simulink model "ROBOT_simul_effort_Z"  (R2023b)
settings: Solver=VariableStepAuto  StartTime=0.0  StopTime=5  RelTol=1e-3
undefined symbols (not defined in the file): deg, kg, m, manette1_Defaut_sldprt, manette2_Defaut_sldprt, mm, N, rad, s, STL, X, Y, Z
libraries: sm_lib x463, fl_lib x45, nesl_utility x27, simulink x2
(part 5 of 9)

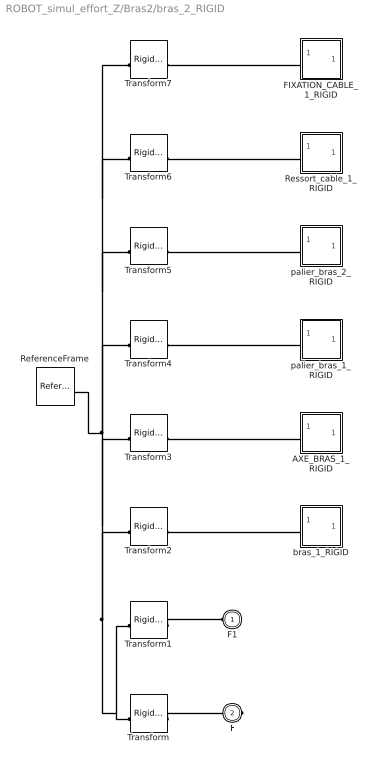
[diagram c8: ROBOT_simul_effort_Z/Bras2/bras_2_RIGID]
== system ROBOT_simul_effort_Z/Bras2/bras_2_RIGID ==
  AXE_BRAS_1_RIGID : Subsystem
  FIXATION_CABLE_1_RIGID : Subsystem
  ReferenceFrame : sm_lib/Frames and Transforms/Reference Frame
  Ressort_cable_1_RIGID : Subsystem
  Transform : sm_lib/Frames and Transforms/Rigid Transform  TranslationMethod=Cartesian  TranslationStandardOffset=0  TranslationStandardOffsetUnits=mm  TranslationStandardAxis=+Z  TranslationCartesianOffset=[-176.59192436800635 99.825618202078147 -20.98098974470366]  TranslationCartesianOffsetUnits=mm  TranslationROffset=0  TranslationROffsetUnits=m  TranslationZOffset=0  TranslationZOffsetUnits=m  TranslationThetaOffset=0  TranslationThetaOffsetUnits=deg  RotationMethod=ArbitraryAxis  RotationAngleUnits=rad  RotationStandardAxis=+Z  RotationAngle=2.0943951023931953  RotationArbitraryAxis=[0.57735026918962584 0.57735026918962562 0.57735026918962584]  FollAlignAxisA=+X  BaseAlignAxisA=+Y  FollAlignAxisB=+Y  BaseAlignAxisB=+Z  RotationSequenceAxes=FollowerAxes  RotationSequence=XYX  RotationSequenceAngles=[0 0 0]  RotationSequenceAnglesUnits=deg  RotationMatrix=[1 0 0; 0 1 0; 0 0 1]  Quaternion=[1 0 0 0]
  Transform1 : sm_lib/Frames and Transforms/Rigid Transform  TranslationMethod=Cartesian  TranslationStandardOffset=0  TranslationStandardOffsetUnits=mm  TranslationStandardAxis=+Z  TranslationCartesianOffset=[-252.36832285678628 39.825618202076186 -20.980989744713362]  TranslationCartesianOffsetUnits=mm  TranslationROffset=0  TranslationROffsetUnits=m  TranslationZOffset=0  TranslationZOffsetUnits=m  TranslationThetaOffset=0  TranslationThetaOffsetUnits=deg  RotationMethod=ArbitraryAxis  RotationAngleUnits=rad  RotationStandardAxis=+Z  RotationAngle=2.0943951023931948  RotationArbitraryAxis=[0.57735026918962573 0.57735026918962562 0.57735026918962595]  FollAlignAxisA=+X  BaseAlignAxisA=+Y  FollAlignAxisB=+Y  BaseAlignAxisB=+Z  RotationSequenceAxes=FollowerAxes  RotationSequence=XYX  RotationSequenceAngles=[0 0 0]  RotationSequenceAnglesUnits=deg  RotationMatrix=[1 0 0; 0 1 0; 0 0 1]  Quaternion=[1 0 0 0]
  Transform2 : sm_lib/Frames and Transforms/Rigid Transform  TranslationMethod=Cartesian  TranslationStandardOffset=0  TranslationStandardOffsetUnits=mm  TranslationStandardAxis=+Z  TranslationCartesianOffset=[-166.59192436800635 39.825618202078161 -20.98098974470367]  TranslationCartesianOffsetUnits=mm  TranslationROffset=0  TranslationROffsetUnits=m  TranslationZOffset=0  TranslationZOffsetUnits=m  TranslationThetaOffset=0  TranslationThetaOffsetUnits=deg  RotationMethod=ArbitraryAxis  RotationAngleUnits=rad  RotationStandardAxis=+Z  RotationAngle=1.5707963267948968  RotationArbitraryAxis=[9.841111005584301e-17 -1 -9.841111005584301e-17]  FollAlignAxisA=+X  BaseAlignAxisA=+Y  FollAlignAxisB=+Y  BaseAlignAxisB=+Z  RotationSequenceAxes=FollowerAxes  RotationSequence=XYX  RotationSequenceAngles=[0 0 0]  RotationSequenceAnglesUnits=deg  RotationMatrix=[1 0 0; 0 1 0; 0 0 1]  Quaternion=[1 0 0 0]
  Transform3 : sm_lib/Frames and Transforms/Rigid Transform  TranslationMethod=Cartesian  TranslationStandardOffset=0  TranslationStandardOffsetUnits=mm  TranslationStandardAxis=+Z  TranslationCartesianOffset=[-166.59192436800635 39.825618202078161 -20.98098974470367]  TranslationCartesianOffsetUnits=mm  TranslationROffset=0  TranslationROffsetUnits=m  TranslationZOffset=0  TranslationZOffsetUnits=m  TranslationThetaOffset=0  TranslationThetaOffsetUnits=deg  RotationMethod=ArbitraryAxis  RotationAngleUnits=rad  RotationStandardAxis=+Z  RotationAngle=1.5707963267948968  RotationArbitraryAxis=[-9.841111005584301e-17 1 -9.841111005584301e-17]  FollAlignAxisA=+X  BaseAlignAxisA=+Y  FollAlignAxisB=+Y  BaseAlignAxisB=+Z  RotationSequenceAxes=FollowerAxes  RotationSequence=XYX  RotationSequenceAngles=[0 0 0]  RotationSequenceAnglesUnits=deg  RotationMatrix=[1 0 0; 0 1 0; 0 0 1]  Quaternion=[1 0 0 0]
  Transform4 : sm_lib/Frames and Transforms/Rigid Transform  TranslationMethod=None  TranslationStandardOffset=0  TranslationStandardOffsetUnits=m  TranslationStandardAxis=+Z  TranslationCartesianOffset=[0 0 0]  TranslationCartesianOffsetUnits=m  TranslationROffset=0  TranslationROffsetUnits=m  TranslationZOffset=0  TranslationZOffsetUnits=m  TranslationThetaOffset=0  TranslationThetaOffsetUnits=deg  RotationMethod=None  RotationAngleUnits=deg  RotationStandardAxis=+Z  RotationAngle=0  RotationArbitraryAxis=[0 0 1]  FollAlignAxisA=+X  BaseAlignAxisA=+Y  FollAlignAxisB=+Y  BaseAlignAxisB=+Z  RotationSequenceAxes=FollowerAxes  RotationSequence=XYX  RotationSequenceAngles=[0 0 0]  RotationSequenceAnglesUnits=deg  RotationMatrix=[1 0 0; 0 1 0; 0 0 1]  Quaternion=[1 0 0 0]
  Transform5 : sm_lib/Frames and Transforms/Rigid Transform  TranslationMethod=Cartesian  TranslationStandardOffset=0  TranslationStandardOffsetUnits=mm  TranslationStandardAxis=+Z  TranslationCartesianOffset=[-333.18384873601269 5.2270863233389981 7.8152493791980318]  TranslationCartesianOffsetUnits=mm  TranslationROffset=0  TranslationROffsetUnits=m  TranslationZOffset=0  TranslationZOffsetUnits=m  TranslationThetaOffset=0  TranslationThetaOffsetUnits=deg  RotationMethod=ArbitraryAxis  RotationAngleUnits=rad  RotationStandardAxis=+Z  RotationAngle=3.1415926535897931  RotationArbitraryAxis=[5.9196876012963212e-17 0.83121877946981937 -0.55594544755461739]  FollAlignAxisA=+X  BaseAlignAxisA=+Y  FollAlignAxisB=+Y  BaseAlignAxisB=+Z  RotationSequenceAxes=FollowerAxes  RotationSequence=XYX  RotationSequenceAngles=[0 0 0]  RotationSequenceAnglesUnits=deg  RotationMatrix=[1 0 0; 0 1 0; 0 0 1]  Quaternion=[1 0 0 0]
  Transform6 : sm_lib/Frames and Transforms/Rigid Transform  TranslationMethod=Cartesian  TranslationStandardOffset=0  TranslationStandardOffsetUnits=mm  TranslationStandardAxis=+Z  TranslationCartesianOffset=[-166.59192436800635 17.1829411352671 -24.980989744703674]  TranslationCartesianOffsetUnits=mm  TranslationROffset=0  TranslationROffsetUnits=m  TranslationZOffset=0  TranslationZOffsetUnits=m  TranslationThetaOffset=0  TranslationThetaOffsetUnits=deg  RotationMethod=ArbitraryAxis  RotationAngleUnits=rad  RotationStandardAxis=+Z  RotationAngle=1.5707963267948968  RotationArbitraryAxis=[1 -9.841111005584301e-17 9.8411110055842801e-17]  FollAlignAxisA=+X  BaseAlignAxisA=+Y  FollAlignAxisB=+Y  BaseAlignAxisB=+Z  RotationSequenceAxes=FollowerAxes  RotationSequence=XYX  RotationSequenceAngles=[0 0 0]  RotationSequenceAnglesUnits=deg  RotationMatrix=[1 0 0; 0 1 0; 0 0 1]  Quaternion=[1 0 0 0]
  Transform7 : sm_lib/Frames and Transforms/Rigid Transform  TranslationMethod=Cartesian  TranslationStandardOffset=0  TranslationStandardOffsetUnits=mm  TranslationStandardAxis=+Z  TranslationCartesianOffset=[-172.59192436800635 90.586314327933934 3.4188407632840172]  TranslationCartesianOffsetUnits=mm  TranslationROffset=0  TranslationROffsetUnits=m  TranslationZOffset=0  TranslationZOffsetUnits=m  TranslationThetaOffset=0  TranslationThetaOffsetUnits=deg  RotationMethod=ArbitraryAxis  RotationAngleUnits=rad  RotationStandardAxis=+Z  RotationAngle=1.0159852938148253  RotationArbitraryAxis=[-1 0 -1.1577777653628589e-16]  FollAlignAxisA=+X  BaseAlignAxisA=+Y  FollAlignAxisB=+Y  BaseAlignAxisB=+Z  RotationSequenceAxes=FollowerAxes  RotationSequence=XYX  RotationSequenceAngles=[0 0 0]  RotationSequenceAnglesUnits=deg  RotationMatrix=[1 0 0; 0 1 0; 0 0 1]  Quaternion=[1 0 0 0]
  bras_1_RIGID : Subsystem
  palier_bras_1_RIGID : Subsystem
  palier_bras_2_RIGID : Subsystem
  F1 : PMIOPort  Side=Left
  F : PMIOPort  Port=2  Side=Right
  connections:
  Transform/LConn1 -- ReferenceFrame/RConn1 -- Transform6/LConn1 -- Transform7/LConn1 -- Transform5/LConn1 -- Transform4/LConn1 -- Transform3/LConn1 -- Transform2/LConn1 -- Transform1/LConn1
  Transform/RConn1 -- F/RConn1
  Transform1/RConn1 -- F1/RConn1
  Transform2/RConn1 -- bras_1_RIGID/LConn1
  AXE_BRAS_1_RIGID/LConn1 -- Transform3/RConn1
  Transform4/RConn1 -- palier_bras_1_RIGID/LConn1
  Transform5/RConn1 -- palier_bras_2_RIGID/LConn1
  Ressort_cable_1_RIGID/LConn1 -- Transform6/RConn1
  FIXATION_CABLE_1_RIGID/LConn1 -- Transform7/RConn1

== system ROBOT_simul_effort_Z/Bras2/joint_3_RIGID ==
  AXE_BRAS_1_RIGID : Subsystem
  ReferenceFrame : sm_lib/Frames and Transforms/Reference Frame
  Transform : sm_lib/Frames and Transforms/Rigid Transform  TranslationMethod=Cartesian  TranslationStandardOffset=0  TranslationStandardOffsetUnits=mm  TranslationStandardAxis=+Z  TranslationCartesianOffset=[-182.62772197331239 126.3991346976174 -143.1183707091507]  TranslationCartesianOffsetUnits=mm  TranslationROffset=0  TranslationROffsetUnits=m  TranslationZOffset=0  TranslationZOffsetUnits=m  TranslationThetaOffset=0  TranslationThetaOffsetUnits=deg  RotationMethod=ArbitraryAxis  RotationAngleUnits=rad  RotationStandardAxis=+Z  RotationAngle=2.0943951023931953  RotationArbitraryAxis=[0.57735026918962584 0.57735026918962584 0.57735026918962584]  FollAlignAxisA=+X  BaseAlignAxisA=+Y  FollAlignAxisB=+Y  BaseAlignAxisB=+Z  RotationSequenceAxes=FollowerAxes  RotationSequence=XYX  RotationSequenceAngles=[0 0 0]  RotationSequenceAnglesUnits=deg  RotationMatrix=[1 0 0; 0 1 0; 0 0 1]  Quaternion=[1 0 0 0]
  Transform1 : sm_lib/Frames and Transforms/Rigid Transform  TranslationMethod=Cartesian  TranslationStandardOffset=0  TranslationStandardOffsetUnits=mm  TranslationStandardAxis=+Z  TranslationCartesianOffset=[-181.62772197331239 116.1902983931664 -133.8263224253264]  TranslationCartesianOffsetUnits=mm  TranslationROffset=0  TranslationROffsetUnits=m  TranslationZOffset=0  TranslationZOffsetUnits=m  TranslationThetaOffset=0  TranslationThetaOffsetUnits=deg  RotationMethod=ArbitraryAxis  RotationAngleUnits=rad  RotationStandardAxis=+Z  RotationAngle=1.9754511492118267  RotationArbitraryAxis=[-0.53149434051907762 -0.5314943405190774 -0.65956616953296032]  FollAlignAxisA=+X  BaseAlignAxisA=+Y  FollAlignAxisB=+Y  BaseAlignAxisB=+Z  RotationSequenceAxes=FollowerAxes  RotationSequence=XYX  RotationSequenceAngles=[0 0 0]  RotationSequenceAnglesUnits=deg  RotationMatrix=[1 0 0; 0 1 0; 0 0 1]  Quaternion=[1 0 0 0]
  Transform2 : sm_lib/Frames and Transforms/Rigid Transform  TranslationMethod=Cartesian  TranslationStandardOffset=0  TranslationStandardOffsetUnits=mm  TranslationStandardAxis=+Z  TranslationCartesianOffset=[-153.62772197331239 116.19029839316639 -133.82632242532642]  TranslationCartesianOffsetUnits=mm  TranslationROffset=0  TranslationROffsetUnits=m  TranslationZOffset=0  TranslationZOffsetUnits=m  TranslationThetaOffset=0  TranslationThetaOffsetUnits=deg  RotationMethod=ArbitraryAxis  RotationAngleUnits=rad  RotationStandardAxis=+Z  RotationAngle=1.9754511492118267  RotationArbitraryAxis=[-0.53149434051907762 -0.5314943405190774 -0.65956616953296032]  FollAlignAxisA=+X  BaseAlignAxisA=+Y  FollAlignAxisB=+Y  BaseAlignAxisB=+Z  RotationSequenceAxes=FollowerAxes  RotationSequence=XYX  RotationSequenceAngles=[0 0 0]  RotationSequenceAnglesUnits=deg  RotationMatrix=[1 0 0; 0 1 0; 0 0 1]  Quaternion=[1 0 0 0]
  Transform3 : sm_lib/Frames and Transforms/Rigid Transform  TranslationMethod=Cartesian  TranslationStandardOffset=0  TranslationStandardOffsetUnits=mm  TranslationStandardAxis=+Z  TranslationCartesianOffset=[-167.62772197331242 128.09991096385988 -150.93549038919826]  TranslationCartesianOffsetUnits=mm  TranslationROffset=0  TranslationROffsetUnits=m  TranslationZOffset=0  TranslationZOffsetUnits=m  TranslationThetaOffset=0  TranslationThetaOffsetUnits=deg  RotationMethod=ArbitraryAxis  RotationAngleUnits=rad  RotationStandardAxis=+Z  RotationAngle=1.7850283121554718  RotationArbitraryAxis=[1 6.7005179906918671e-16 -7.8797744802439854e-16]  FollAlignAxisA=+X  BaseAlignAxisA=+Y  FollAlignAxisB=+Y  BaseAlignAxisB=+Z  RotationSequenceAxes=FollowerAxes  RotationSequence=XYX  RotationSequenceAngles=[0 0 0]  RotationSequenceAnglesUnits=deg  RotationMatrix=[1 0 0; 0 1 0; 0 0 1]  Quaternion=[1 0 0 0]
  Transform4 : sm_lib/Frames and Transforms/Rigid Transform  TranslationMethod=Cartesian  TranslationStandardOffset=0  TranslationStandardOffsetUnits=mm  TranslationStandardAxis=+Z  TranslationCartesianOffset=[-167.62772197331239 126.3991346976174 -143.1183707091507]  TranslationCartesianOffsetUnits=mm  TranslationROffset=0  TranslationROffsetUnits=m  TranslationZOffset=0  TranslationZOffsetUnits=m  TranslationThetaOffset=0  TranslationThetaOffsetUnits=deg  RotationMethod=ArbitraryAxis  RotationAngleUnits=rad  RotationStandardAxis=+Z  RotationAngle=1.5707963267948968  RotationArbitraryAxis=[8.0498418078381935e-17 -1 8.0498418078381935e-17]  FollAlignAxisA=+X  BaseAlignAxisA=+Y  FollAlignAxisB=+Y  BaseAlignAxisB=+Z  RotationSequenceAxes=FollowerAxes  RotationSequence=XYX  RotationSequenceAngles=[0 0 0]  RotationSequenceAnglesUnits=deg  RotationMatrix=[1 0 0; 0 1 0; 0 0 1]  Quaternion=[1 0 0 0]
  joint_1_RIGID : Subsystem
  F2 : PMIOPort  Side=Left
  F : PMIOPort  Port=2  Side=Right
  F1 : PMIOPort  Port=3  Side=Left
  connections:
  Transform/LConn1 -- ReferenceFrame/RConn1 -- Transform3/LConn1 -- Transform4/LConn1 -- Transform2/LConn1 -- Transform1/LConn1
  Transform/RConn1 -- F/RConn1
  Transform1/RConn1 -- F1/RConn1
  Transform2/RConn1 -- F2/RConn1
  Transform3/RConn1 -- joint_1_RIGID/LConn1
  AXE_BRAS_1_RIGID/LConn1 -- Transform4/RConn1

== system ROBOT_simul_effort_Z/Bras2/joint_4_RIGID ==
  AXE_BRAS_1_RIGID : Subsystem
  ReferenceFrame : sm_lib/Frames and Transforms/Reference Frame
  Transform : sm_lib/Frames and Transforms/Rigid Transform  TranslationMethod=Cartesian  TranslationStandardOffset=0  TranslationStandardOffsetUnits=mm  TranslationStandardAxis=+Z  TranslationCartesianOffset=[-177.62772197331228 126.39913469764599 -143.11837070916687]  TranslationCartesianOffsetUnits=mm  TranslationROffset=0  TranslationROffsetUnits=m  TranslationZOffset=0  TranslationZOffsetUnits=m  TranslationThetaOffset=0  TranslationThetaOffsetUnits=deg  RotationMethod=ArbitraryAxis  RotationAngleUnits=rad  RotationStandardAxis=+Z  RotationAngle=2.0943951023931962  RotationArbitraryAxis=[0.5773502691896254 0.57735026918962584 0.57735026918962595]  FollAlignAxisA=+X  BaseAlignAxisA=+Y  FollAlignAxisB=+Y  BaseAlignAxisB=+Z  RotationSequenceAxes=FollowerAxes  RotationSequence=XYX  RotationSequenceAngles=[0 0 0]  RotationSequenceAnglesUnits=deg  RotationMatrix=[1 0 0; 0 1 0; 0 0 1]  Quaternion=[1 0 0 0]
  Transform1 : sm_lib/Frames and Transforms/Rigid Transform  TranslationMethod=Cartesian  TranslationStandardOffset=0  TranslationStandardOffsetUnits=mm  TranslationStandardAxis=+Z  TranslationCartesianOffset=[-181.6277219733183 116.19029839316549 -133.82632242532227]  TranslationCartesianOffsetUnits=mm  TranslationROffset=0  TranslationROffsetUnits=m  TranslationZOffset=0  TranslationZOffsetUnits=m  TranslationThetaOffset=0  TranslationThetaOffsetUnits=deg  RotationMethod=ArbitraryAxis  RotationAngleUnits=rad  RotationStandardAxis=+Z  RotationAngle=1.9754511492118263  RotationArbitraryAxis=[-0.53149434051907762 -0.53149434051907762 -0.6595661695329601]  FollAlignAxisA=+X  BaseAlignAxisA=+Y  FollAlignAxisB=+Y  BaseAlignAxisB=+Z  RotationSequenceAxes=FollowerAxes  RotationSequence=XYX  RotationSequenceAngles=[0 0 0]  RotationSequenceAnglesUnits=deg  RotationMatrix=[1 0 0; 0 1 0; 0 0 1]  Quaternion=[1 0 0 0]
  Transform2 : sm_lib/Frames and Transforms/Rigid Transform  TranslationMethod=Cartesian  TranslationStandardOffset=0  TranslationStandardOffsetUnits=mm  TranslationStandardAxis=+Z  TranslationCartesianOffset=[-153.62772197331839 131.82453775326127 -130.42476989284023]  TranslationCartesianOffsetUnits=mm  TranslationROffset=0  TranslationROffsetUnits=m  TranslationZOffset=0  TranslationZOffsetUnits=m  TranslationThetaOffset=0  TranslationThetaOffsetUnits=deg  RotationMethod=ArbitraryAxis  RotationAngleUnits=rad  RotationStandardAxis=+Z  RotationAngle=2.2221940470110662  RotationArbitraryAxis=[0.61437017396792992 -0.61437017396793137 0.49507431631748922]  FollAlignAxisA=+X  BaseAlignAxisA=+Y  FollAlignAxisB=+Y  BaseAlignAxisB=+Z  RotationSequenceAxes=FollowerAxes  RotationSequence=XYX  RotationSequenceAngles=[0 0 0]  RotationSequenceAnglesUnits=deg  RotationMatrix=[1 0 0; 0 1 0; 0 0 1]  Quaternion=[1 0 0 0]
  Transform3 : sm_lib/Frames and Transforms/Rigid Transform  TranslationMethod=Cartesian  TranslationStandardOffset=0  TranslationStandardOffsetUnits=mm  TranslationStandardAxis=+Z  TranslationCartesianOffset=[-167.62772197331242 128.09991096385986 -150.93549038919815]  TranslationCartesianOffsetUnits=mm  TranslationROffset=0  TranslationROffsetUnits=m  TranslationZOffset=0  TranslationZOffsetUnits=m  TranslationThetaOffset=0  TranslationThetaOffsetUnits=deg  RotationMethod=ArbitraryAxis  RotationAngleUnits=rad  RotationStandardAxis=+Z  RotationAngle=1.785028312155472  RotationArbitraryAxis=[1 8.8696087027513098e-16 -7.493533857789905e-16]  FollAlignAxisA=+X  BaseAlignAxisA=+Y  FollAlignAxisB=+Y  BaseAlignAxisB=+Z  RotationSequenceAxes=FollowerAxes  RotationSequence=XYX  RotationSequenceAngles=[0 0 0]  RotationSequenceAnglesUnits=deg  RotationMatrix=[1 0 0; 0 1 0; 0 0 1]  Quaternion=[1 0 0 0]
  Transform4 : sm_lib/Frames and Transforms/Rigid Transform  TranslationMethod=Cartesian  TranslationStandardOffset=0  TranslationStandardOffsetUnits=mm  TranslationStandardAxis=+Z  TranslationCartesianOffset=[-167.62772197331239 126.39913469761737 -143.11837070915061]  TranslationCartesianOffsetUnits=mm  TranslationROffset=0  TranslationROffsetUnits=m  TranslationZOffset=0  TranslationZOffsetUnits=m  TranslationThetaOffset=0  TranslationThetaOffsetUnits=deg  RotationMethod=ArbitraryAxis  RotationAngleUnits=rad  RotationStandardAxis=+Z  RotationAngle=1.570796326794897  RotationArbitraryAxis=[-0 -1 -0]  FollAlignAxisA=+X  BaseAlignAxisA=+Y  FollAlignAxisB=+Y  BaseAlignAxisB=+Z  RotationSequenceAxes=FollowerAxes  RotationSequence=XYX  RotationSequenceAngles=[0 0 0]  RotationSequenceAnglesUnits=deg  RotationMatrix=[1 0 0; 0 1 0; 0 0 1]  Quaternion=[1 0 0 0]
  joint_1_RIGID : Subsystem
  F2 : PMIOPort  Side=Right
  F1 : PMIOPort  Port=2  Side=Right
  F : PMIOPort  Port=3  Side=Left
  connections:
  Transform/LConn1 -- ReferenceFrame/RConn1 -- Transform3/LConn1 -- Transform4/LConn1 -- Transform2/LConn1 -- Transform1/LConn1
  Transform/RConn1 -- F/RConn1
  Transform1/RConn1 -- F1/RConn1
  Transform2/RConn1 -- F2/RConn1
  Transform3/RConn1 -- joint_1_RIGID/LConn1
  AXE_BRAS_1_RIGID/LConn1 -- Transform4/RConn1

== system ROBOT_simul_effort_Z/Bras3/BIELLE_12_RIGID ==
  AXE_BIELLE_1_RIGID : Subsystem
  AXE_BIELLE_2_RIGID : Subsystem
  BIELLE_PARALLELOGRAMME_1_RIGID : Subsystem
  ReferenceFrame : sm_lib/Frames and Transforms/Reference Frame
  Transform : sm_lib/Frames and Transforms/Rigid Transform  TranslationMethod=Cartesian  TranslationStandardOffset=0  TranslationStandardOffsetUnits=mm  TranslationStandardAxis=+Z  TranslationCartesianOffset=[-181.12877100136717 12.999999999999996 -3.249999999999996]  TranslationCartesianOffsetUnits=mm  TranslationROffset=0  TranslationROffsetUnits=m  TranslationZOffset=0  TranslationZOffsetUnits=m  TranslationThetaOffset=0  TranslationThetaOffsetUnits=deg  RotationMethod=ArbitraryAxis  RotationAngleUnits=rad  RotationStandardAxis=+Z  RotationAngle=2.0943951023931953  RotationArbitraryAxis=[0.57735026918962584 -0.57735026918962584 0.57735026918962584]  FollAlignAxisA=+X  BaseAlignAxisA=+Y  FollAlignAxisB=+Y  BaseAlignAxisB=+Z  RotationSequenceAxes=FollowerAxes  RotationSequence=XYX  RotationSequenceAngles=[0 0 0]  RotationSequenceAnglesUnits=deg  RotationMatrix=[1 0 0; 0 1 0; 0 0 1]  Quaternion=[1 0 0 0]
  Transform1 : sm_lib/Frames and Transforms/Rigid Transform  TranslationMethod=Cartesian  TranslationStandardOffset=0  TranslationStandardOffsetUnits=mm  TranslationStandardAxis=+Z  TranslationCartesianOffset=[-181.1287710013672 12.999999999999963 -105.75000000000004]  TranslationCartesianOffsetUnits=mm  TranslationROffset=0  TranslationROffsetUnits=m  TranslationZOffset=0  TranslationZOffsetUnits=m  TranslationThetaOffset=0  TranslationThetaOffsetUnits=deg  RotationMethod=ArbitraryAxis  RotationAngleUnits=rad  RotationStandardAxis=+Z  RotationAngle=2.0943951023931957  RotationArbitraryAxis=[0.57735026918962573 -0.57735026918962573 0.57735026918962562]  FollAlignAxisA=+X  BaseAlignAxisA=+Y  FollAlignAxisB=+Y  BaseAlignAxisB=+Z  RotationSequenceAxes=FollowerAxes  RotationSequence=XYX  RotationSequenceAngles=[0 0 0]  RotationSequenceAnglesUnits=deg  RotationMatrix=[1 0 0; 0 1 0; 0 0 1]  Quaternion=[1 0 0 0]
  Transform2 : sm_lib/Frames and Transforms/Rigid Transform  TranslationMethod=Cartesian  TranslationStandardOffset=0  TranslationStandardOffsetUnits=mm  TranslationStandardAxis=+Z  TranslationCartesianOffset=[-178.12877100136717 4.9999999999999902 -54.500000000000021]  TranslationCartesianOffsetUnits=mm  TranslationROffset=0  TranslationROffsetUnits=m  TranslationZOffset=0  TranslationZOffsetUnits=m  TranslationThetaOffset=0  TranslationThetaOffsetUnits=deg  RotationMethod=ArbitraryAxis  RotationAngleUnits=rad  RotationStandardAxis=+Z  RotationAngle=3.1415926535897931  RotationArbitraryAxis=[-0.70710678118654746 0.70710678118654757 0]  FollAlignAxisA=+X  BaseAlignAxisA=+Y  FollAlignAxisB=+Y  BaseAlignAxisB=+Z  RotationSequenceAxes=FollowerAxes  RotationSequence=XYX  RotationSequenceAngles=[0 0 0]  RotationSequenceAnglesUnits=deg  RotationMatrix=[1 0 0; 0 1 0; 0 0 1]  Quaternion=[1 0 0 0]
  Transform3 : sm_lib/Frames and Transforms/Rigid Transform  TranslationMethod=Cartesian  TranslationStandardOffset=0  TranslationStandardOffsetUnits=mm  TranslationStandardAxis=+Z  TranslationCartesianOffset=[-181.1287710013672 4.9999999999999627 -105.75000000000004]  TranslationCartesianOffsetUnits=mm  TranslationROffset=0  TranslationROffsetUnits=m  TranslationZOffset=0  TranslationZOffsetUnits=m  TranslationThetaOffset=0  TranslationThetaOffsetUnits=deg  RotationMethod=ArbitraryAxis  RotationAngleUnits=rad  RotationStandardAxis=+Z  RotationAngle=1.7602050674842991  RotationArbitraryAxis=[-0.82650316451596495 -0.39805308631204944 -0.39805308631204944]  FollAlignAxisA=+X  BaseAlignAxisA=+Y  FollAlignAxisB=+Y  BaseAlignAxisB=+Z  RotationSequenceAxes=FollowerAxes  RotationSequence=XYX  RotationSequenceAngles=[0 0 0]  RotationSequenceAnglesUnits=deg  RotationMatrix=[1 0 0; 0 1 0; 0 0 1]  Quaternion=[1 0 0 0]
  Transform4 : sm_lib/Frames and Transforms/Rigid Transform  TranslationMethod=Cartesian  TranslationStandardOffset=0  TranslationStandardOffsetUnits=mm  TranslationStandardAxis=+Z  TranslationCartesianOffset=[-181.12877100136717 4.9999999999999902 -3.249999999999996]  TranslationCartesianOffsetUnits=mm  TranslationROffset=0  TranslationROffsetUnits=m  TranslationZOffset=0  TranslationZOffsetUnits=m  TranslationThetaOffset=0  TranslationThetaOffsetUnits=deg  RotationMethod=ArbitraryAxis  RotationAngleUnits=rad  RotationStandardAxis=+Z  RotationAngle=1.7602050674842997  RotationArbitraryAxis=[-0.82650316451596506 -0.39805308631204933 -0.39805308631204939]  FollAlignAxisA=+X  BaseAlignAxisA=+Y  FollAlignAxisB=+Y  BaseAlignAxisB=+Z  RotationSequenceAxes=FollowerAxes  RotationSequence=XYX  RotationSequenceAngles=[0 0 0]  RotationSequenceAnglesUnits=deg  RotationMatrix=[1 0 0; 0 1 0; 0 0 1]  Quaternion=[1 0 0 0]
  F1 : PMIOPort  Side=Left
  F : PMIOPort  Port=2  Side=Right
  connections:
  Transform/LConn1 -- ReferenceFrame/RConn1 -- Transform3/LConn1 -- Transform4/LConn1 -- Transform2/LConn1 -- Transform1/LConn1
  Transform/RConn1 -- F/RConn1
  Transform1/RConn1 -- F1/RConn1
  BIELLE_PARALLELOGRAMME_1_RIGID/LConn1 -- Transform2/RConn1
  AXE_BIELLE_1_RIGID/LConn1 -- Transform3/RConn1
  AXE_BIELLE_2_RIGID/LConn1 -- Transform4/RConn1

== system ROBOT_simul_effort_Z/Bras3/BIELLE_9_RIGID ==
  AXE_BIELLE_1_RIGID : Subsystem
  AXE_BIELLE_2_RIGID : Subsystem
  BIELLE_PARALLELOGRAMME_1_RIGID : Subsystem
  ReferenceFrame : sm_lib/Frames and Transforms/Reference Frame
  Transform : sm_lib/Frames and Transforms/Rigid Transform  TranslationMethod=Cartesian  TranslationStandardOffset=0  TranslationStandardOffsetUnits=mm  TranslationStandardAxis=+Z  TranslationCartesianOffset=[-181.12877100136723 12.999999999999982 -105.75000000000001]  TranslationCartesianOffsetUnits=mm  TranslationROffset=0  TranslationROffsetUnits=m  TranslationZOffset=0  TranslationZOffsetUnits=m  TranslationThetaOffset=0  TranslationThetaOffsetUnits=deg  RotationMethod=ArbitraryAxis  RotationAngleUnits=rad  RotationStandardAxis=+Z  RotationAngle=2.0943951023931957  RotationArbitraryAxis=[0.57735026918962573 -0.57735026918962573 0.57735026918962562]  FollAlignAxisA=+X  BaseAlignAxisA=+Y  FollAlignAxisB=+Y  BaseAlignAxisB=+Z  RotationSequenceAxes=FollowerAxes  RotationSequence=XYX  RotationSequenceAngles=[0 0 0]  RotationSequenceAnglesUnits=deg  RotationMatrix=[1 0 0; 0 1 0; 0 0 1]  Quaternion=[1 0 0 0]
  Transform1 : sm_lib/Frames and Transforms/Rigid Transform  TranslationMethod=Cartesian  TranslationStandardOffset=0  TranslationStandardOffsetUnits=mm  TranslationStandardAxis=+Z  TranslationCartesianOffset=[-181.12877100136717 13.000000000000004 -3.2500000000000151]  TranslationCartesianOffsetUnits=mm  TranslationROffset=0  TranslationROffsetUnits=m  TranslationZOffset=0  TranslationZOffsetUnits=m  TranslationThetaOffset=0  TranslationThetaOffsetUnits=deg  RotationMethod=ArbitraryAxis  RotationAngleUnits=rad  RotationStandardAxis=+Z  RotationAngle=2.0943951023931957  RotationArbitraryAxis=[0.57735026918962584 -0.57735026918962573 0.57735026918962573]  FollAlignAxisA=+X  BaseAlignAxisA=+Y  FollAlignAxisB=+Y  BaseAlignAxisB=+Z  RotationSequenceAxes=FollowerAxes  RotationSequence=XYX  RotationSequenceAngles=[0 0 0]  RotationSequenceAnglesUnits=deg  RotationMatrix=[1 0 0; 0 1 0; 0 0 1]  Quaternion=[1 0 0 0]
  Transform2 : sm_lib/Frames and Transforms/Rigid Transform  TranslationMethod=Cartesian  TranslationStandardOffset=0  TranslationStandardOffsetUnits=mm  TranslationStandardAxis=+Z  TranslationCartesianOffset=[-178.12877100136717 5.0000000000000044 -54.500000000000021]  TranslationCartesianOffsetUnits=mm  TranslationROffset=0  TranslationROffsetUnits=m  TranslationZOffset=0  TranslationZOffsetUnits=m  TranslationThetaOffset=0  TranslationThetaOffsetUnits=deg  RotationMethod=ArbitraryAxis  RotationAngleUnits=rad  RotationStandardAxis=+Z  RotationAngle=3.1415926535897931  RotationArbitraryAxis=[0.70710678118654746 -0.70710678118654757 3.9252311467094379e-17]  FollAlignAxisA=+X  BaseAlignAxisA=+Y  FollAlignAxisB=+Y  BaseAlignAxisB=+Z  RotationSequenceAxes=FollowerAxes  RotationSequence=XYX  RotationSequenceAngles=[0 0 0]  RotationSequenceAnglesUnits=deg  RotationMatrix=[1 0 0; 0 1 0; 0 0 1]  Quaternion=[1 0 0 0]
  Transform3 : sm_lib/Frames and Transforms/Rigid Transform  TranslationMethod=Cartesian  TranslationStandardOffset=0  TranslationStandardOffsetUnits=mm  TranslationStandardAxis=+Z  TranslationCartesianOffset=[-181.12877100136723 4.9999999999999902 -105.75000000000001]  TranslationCartesianOffsetUnits=mm  TranslationROffset=0  TranslationROffsetUnits=m  TranslationZOffset=0  TranslationZOffsetUnits=m  TranslationThetaOffset=0  TranslationThetaOffsetUnits=deg  RotationMethod=ArbitraryAxis  RotationAngleUnits=rad  RotationStandardAxis=+Z  RotationAngle=1.7602050674842991  RotationArbitraryAxis=[-0.82650316451596495 -0.39805308631204944 -0.39805308631204944]  FollAlignAxisA=+X  BaseAlignAxisA=+Y  FollAlignAxisB=+Y  BaseAlignAxisB=+Z  RotationSequenceAxes=FollowerAxes  RotationSequence=XYX  RotationSequenceAngles=[0 0 0]  RotationSequenceAnglesUnits=deg  RotationMatrix=[1 0 0; 0 1 0; 0 0 1]  Quaternion=[1 0 0 0]
  Transform4 : sm_lib/Frames and Transforms/Rigid Transform  TranslationMethod=Cartesian  TranslationStandardOffset=0  TranslationStandardOffsetUnits=mm  TranslationStandardAxis=+Z  TranslationCartesianOffset=[-181.12877100136717 5.0000000000000044 -3.2500000000000169]  TranslationCartesianOffsetUnits=mm  TranslationROffset=0  TranslationROffsetUnits=m  TranslationZOffset=0  TranslationZOffsetUnits=m  TranslationThetaOffset=0  TranslationThetaOffsetUnits=deg  RotationMethod=ArbitraryAxis  RotationAngleUnits=rad  RotationStandardAxis=+Z  RotationAngle=1.7602050674842993  RotationArbitraryAxis=[-0.82650316451596495 -0.39805308631204939 -0.39805308631204939]  FollAlignAxisA=+X  BaseAlignAxisA=+Y  FollAlignAxisB=+Y  BaseAlignAxisB=+Z  RotationSequenceAxes=FollowerAxes  RotationSequence=XYX  RotationSequenceAngles=[0 0 0]  RotationSequenceAnglesUnits=deg  RotationMatrix=[1 0 0; 0 1 0; 0 0 1]  Quaternion=[1 0 0 0]
  F1 : PMIOPort  Side=Left
  F : PMIOPort  Port=2  Side=Right
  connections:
  Transform/LConn1 -- ReferenceFrame/RConn1 -- Transform3/LConn1 -- Transform4/LConn1 -- Transform2/LConn1 -- Transform1/LConn1
  Transform/RConn1 -- F/RConn1
  Transform1/RConn1 -- F1/RConn1
  BIELLE_PARALLELOGRAMME_1_RIGID/LConn1 -- Transform2/RConn1
  AXE_BIELLE_1_RIGID/LConn1 -- Transform3/RConn1
  AXE_BIELLE_2_RIGID/LConn1 -- Transform4/RConn1

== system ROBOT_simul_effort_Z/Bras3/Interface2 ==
  Angular Velocity Source : fl_lib/Mechanical/Mechanical Sources/Ideal Angular Velocity Source
  Torque Sensor : fl_lib/Mechanical/Mechanical Sensors/Ideal Torque Sensor
  C : PMIOPort  Side=Left
  T : PMIOPort  Port=2  Side=Right
  w : PMIOPort  Port=3  Side=Right
  R : PMIOPort  Port=4  Side=Left
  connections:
  R/RConn1 -- Angular Velocity Source/LConn1
  Torque Sensor/LConn1 -- Angular Velocity Source/RConn2
  Torque Sensor/RConn2 -- T/RConn1
  C/RConn1 -- Torque Sensor/RConn1
  Angular Velocity Source/RConn1 -- w/RConn1

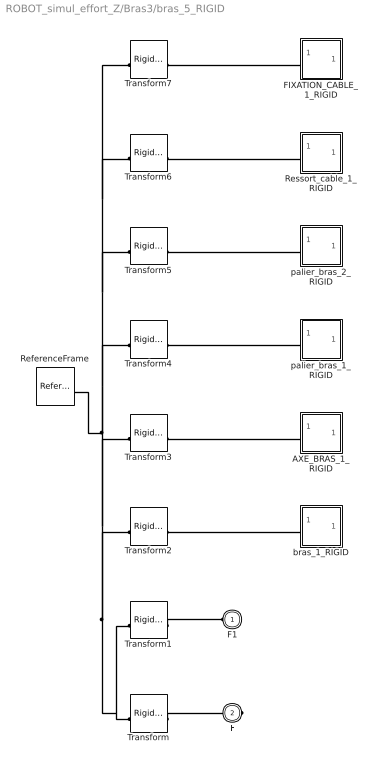
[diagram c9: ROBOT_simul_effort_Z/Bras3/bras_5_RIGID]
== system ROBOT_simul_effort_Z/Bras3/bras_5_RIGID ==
  AXE_BRAS_1_RIGID : Subsystem
  FIXATION_CABLE_1_RIGID : Subsystem
  ReferenceFrame : sm_lib/Frames and Transforms/Reference Frame
  Ressort_cable_1_RIGID : Subsystem
  Transform : sm_lib/Frames and Transforms/Rigid Transform  TranslationMethod=Cartesian  TranslationStandardOffset=0  TranslationStandardOffsetUnits=mm  TranslationStandardAxis=+Z  TranslationCartesianOffset=[-176.59192436800632 99.825618202078189 -20.980989744703674]  TranslationCartesianOffsetUnits=mm  TranslationROffset=0  TranslationROffsetUnits=m  TranslationZOffset=0  TranslationZOffsetUnits=m  TranslationThetaOffset=0  TranslationThetaOffsetUnits=deg  RotationMethod=ArbitraryAxis  RotationAngleUnits=rad  RotationStandardAxis=+Z  RotationAngle=2.0943951023931953  RotationArbitraryAxis=[0.57735026918962584 0.57735026918962584 0.57735026918962584]  FollAlignAxisA=+X  BaseAlignAxisA=+Y  FollAlignAxisB=+Y  BaseAlignAxisB=+Z  RotationSequenceAxes=FollowerAxes  RotationSequence=XYX  RotationSequenceAngles=[0 0 0]  RotationSequenceAnglesUnits=deg  RotationMatrix=[1 0 0; 0 1 0; 0 0 1]  Quaternion=[1 0 0 0]
  Transform1 : sm_lib/Frames and Transforms/Rigid Transform  TranslationMethod=Cartesian  TranslationStandardOffset=0  TranslationStandardOffsetUnits=mm  TranslationStandardAxis=+Z  TranslationCartesianOffset=[-252.36832285678696 39.82561820208025 -20.980989744694625]  TranslationCartesianOffsetUnits=mm  TranslationROffset=0  TranslationROffsetUnits=m  TranslationZOffset=0  TranslationZOffsetUnits=m  TranslationThetaOffset=0  TranslationThetaOffsetUnits=deg  RotationMethod=ArbitraryAxis  RotationAngleUnits=rad  RotationStandardAxis=+Z  RotationAngle=2.0943951023931962  RotationArbitraryAxis=[0.57735026918962562 0.57735026918962595 0.57735026918962573]  FollAlignAxisA=+X  BaseAlignAxisA=+Y  FollAlignAxisB=+Y  BaseAlignAxisB=+Z  RotationSequenceAxes=FollowerAxes  RotationSequence=XYX  RotationSequenceAngles=[0 0 0]  RotationSequenceAnglesUnits=deg  RotationMatrix=[1 0 0; 0 1 0; 0 0 1]  Quaternion=[1 0 0 0]
  Transform2 : sm_lib/Frames and Transforms/Rigid Transform  TranslationMethod=Cartesian  TranslationStandardOffset=0  TranslationStandardOffsetUnits=mm  TranslationStandardAxis=+Z  TranslationCartesianOffset=[-166.59192436800632 39.825618202078182 -20.980989744703674]  TranslationCartesianOffsetUnits=mm  TranslationROffset=0  TranslationROffsetUnits=m  TranslationZOffset=0  TranslationZOffsetUnits=m  TranslationThetaOffset=0  TranslationThetaOffsetUnits=deg  RotationMethod=ArbitraryAxis  RotationAngleUnits=rad  RotationStandardAxis=+Z  RotationAngle=1.5707963267948968  RotationArbitraryAxis=[-0 -1 -0]  FollAlignAxisA=+X  BaseAlignAxisA=+Y  FollAlignAxisB=+Y  BaseAlignAxisB=+Z  RotationSequenceAxes=FollowerAxes  RotationSequence=XYX  RotationSequenceAngles=[0 0 0]  RotationSequenceAnglesUnits=deg  RotationMatrix=[1 0 0; 0 1 0; 0 0 1]  Quaternion=[1 0 0 0]
  Transform3 : sm_lib/Frames and Transforms/Rigid Transform  TranslationMethod=Cartesian  TranslationStandardOffset=0  TranslationStandardOffsetUnits=mm  TranslationStandardAxis=+Z  TranslationCartesianOffset=[-166.59192436800632 39.825618202078182 -20.980989744703674]  TranslationCartesianOffsetUnits=mm  TranslationROffset=0  TranslationROffsetUnits=m  TranslationZOffset=0  TranslationZOffsetUnits=m  TranslationThetaOffset=0  TranslationThetaOffsetUnits=deg  RotationMethod=ArbitraryAxis  RotationAngleUnits=rad  RotationStandardAxis=+Z  RotationAngle=1.5707963267948968  RotationArbitraryAxis=[0 1 0]  FollAlignAxisA=+X  BaseAlignAxisA=+Y  FollAlignAxisB=+Y  BaseAlignAxisB=+Z  RotationSequenceAxes=FollowerAxes  RotationSequence=XYX  RotationSequenceAngles=[0 0 0]  RotationSequenceAnglesUnits=deg  RotationMatrix=[1 0 0; 0 1 0; 0 0 1]  Quaternion=[1 0 0 0]
  Transform4 : sm_lib/Frames and Transforms/Rigid Transform  TranslationMethod=None  TranslationStandardOffset=0  TranslationStandardOffsetUnits=m  TranslationStandardAxis=+Z  TranslationCartesianOffset=[0 0 0]  TranslationCartesianOffsetUnits=m  TranslationROffset=0  TranslationROffsetUnits=m  TranslationZOffset=0  TranslationZOffsetUnits=m  TranslationThetaOffset=0  TranslationThetaOffsetUnits=deg  RotationMethod=None  RotationAngleUnits=deg  RotationStandardAxis=+Z  RotationAngle=0  RotationArbitraryAxis=[0 0 1]  FollAlignAxisA=+X  BaseAlignAxisA=+Y  FollAlignAxisB=+Y  BaseAlignAxisB=+Z  RotationSequenceAxes=FollowerAxes  RotationSequence=XYX  RotationSequenceAngles=[0 0 0]  RotationSequenceAnglesUnits=deg  RotationMatrix=[1 0 0; 0 1 0; 0 0 1]  Quaternion=[1 0 0 0]
  Transform5 : sm_lib/Frames and Transforms/Rigid Transform  TranslationMethod=Cartesian  TranslationStandardOffset=0  TranslationStandardOffsetUnits=mm  TranslationStandardAxis=+Z  TranslationCartesianOffset=[-333.18384873601264 5.2270863233389884 7.8152493791980202]  TranslationCartesianOffsetUnits=mm  TranslationROffset=0  TranslationROffsetUnits=m  TranslationZOffset=0  TranslationZOffsetUnits=m  TranslationThetaOffset=0  TranslationThetaOffsetUnits=deg  RotationMethod=ArbitraryAxis  RotationAngleUnits=rad  RotationStandardAxis=+Z  RotationAngle=3.1415926535897931  RotationArbitraryAxis=[0 0.83121877946981937 -0.55594544755461728]  FollAlignAxisA=+X  BaseAlignAxisA=+Y  FollAlignAxisB=+Y  BaseAlignAxisB=+Z  RotationSequenceAxes=FollowerAxes  RotationSequence=XYX  RotationSequenceAngles=[0 0 0]  RotationSequenceAnglesUnits=deg  RotationMatrix=[1 0 0; 0 1 0; 0 0 1]  Quaternion=[1 0 0 0]
  Transform6 : sm_lib/Frames and Transforms/Rigid Transform  TranslationMethod=Cartesian  TranslationStandardOffset=0  TranslationStandardOffsetUnits=mm  TranslationStandardAxis=+Z  TranslationCartesianOffset=[-166.59192436800629 17.182941135267082 -24.98098974470367]  TranslationCartesianOffsetUnits=mm  TranslationROffset=0  TranslationROffsetUnits=m  TranslationZOffset=0  TranslationZOffsetUnits=m  TranslationThetaOffset=0  TranslationThetaOffsetUnits=deg  RotationMethod=ArbitraryAxis  RotationAngleUnits=rad  RotationStandardAxis=+Z  RotationAngle=1.5707963267948968  RotationArbitraryAxis=[1 0 0]  FollAlignAxisA=+X  BaseAlignAxisA=+Y  FollAlignAxisB=+Y  BaseAlignAxisB=+Z  RotationSequenceAxes=FollowerAxes  RotationSequence=XYX  RotationSequenceAngles=[0 0 0]  RotationSequenceAnglesUnits=deg  RotationMatrix=[1 0 0; 0 1 0; 0 0 1]  Quaternion=[1 0 0 0]
  Transform7 : sm_lib/Frames and Transforms/Rigid Transform  TranslationMethod=Cartesian  TranslationStandardOffset=0  TranslationStandardOffsetUnits=mm  TranslationStandardAxis=+Z  TranslationCartesianOffset=[-172.59192436800629 90.586314327933948 3.4188407632840221]  TranslationCartesianOffsetUnits=mm  TranslationROffset=0  TranslationROffsetUnits=m  TranslationZOffset=0  TranslationZOffsetUnits=m  TranslationThetaOffset=0  TranslationThetaOffsetUnits=deg  RotationMethod=ArbitraryAxis  RotationAngleUnits=rad  RotationStandardAxis=+Z  RotationAngle=1.0159852938148253  RotationArbitraryAxis=[-1 0 0]  FollAlignAxisA=+X  BaseAlignAxisA=+Y  FollAlignAxisB=+Y  BaseAlignAxisB=+Z  RotationSequenceAxes=FollowerAxes  RotationSequence=XYX  RotationSequenceAngles=[0 0 0]  RotationSequenceAnglesUnits=deg  RotationMatrix=[1 0 0; 0 1 0; 0 0 1]  Quaternion=[1 0 0 0]
  bras_1_RIGID : Subsystem
  palier_bras_1_RIGID : Subsystem
  palier_bras_2_RIGID : Subsystem
  F1 : PMIOPort  Side=Left
  F : PMIOPort  Port=2  Side=Right
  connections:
  Transform/LConn1 -- ReferenceFrame/RConn1 -- Transform6/LConn1 -- Transform7/LConn1 -- Transform5/LConn1 -- Transform4/LConn1 -- Transform3/LConn1 -- Transform2/LConn1 -- Transform1/LConn1
  Transform/RConn1 -- F/RConn1
  Transform1/RConn1 -- F1/RConn1
  Transform2/RConn1 -- bras_1_RIGID/LConn1
  AXE_BRAS_1_RIGID/LConn1 -- Transform3/RConn1
  Transform4/RConn1 -- palier_bras_1_RIGID/LConn1
  Transform5/RConn1 -- palier_bras_2_RIGID/LConn1
  Ressort_cable_1_RIGID/LConn1 -- Transform6/RConn1
  FIXATION_CABLE_1_RIGID/LConn1 -- Transform7/RConn1

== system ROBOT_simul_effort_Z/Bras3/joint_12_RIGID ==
  AXE_BRAS_1_RIGID : Subsystem
  ReferenceFrame : sm_lib/Frames and Transforms/Reference Frame
  Transform : sm_lib/Frames and Transforms/Rigid Transform  TranslationMethod=Cartesian  TranslationStandardOffset=0  TranslationStandardOffsetUnits=mm  TranslationStandardAxis=+Z  TranslationCartesianOffset=[-181.62772197331543 131.82453775326098 -130.42476989283941]  TranslationCartesianOffsetUnits=mm  TranslationROffset=0  TranslationROffsetUnits=m  TranslationZOffset=0  TranslationZOffsetUnits=m  TranslationThetaOffset=0  TranslationThetaOffsetUnits=deg  RotationMethod=ArbitraryAxis  RotationAngleUnits=rad  RotationStandardAxis=+Z  RotationAngle=2.2221940470110657  RotationArbitraryAxis=[0.61437017396793003 -0.61437017396793026 0.49507431631749033]  FollAlignAxisA=+X  BaseAlignAxisA=+Y  FollAlignAxisB=+Y  BaseAlignAxisB=+Z  RotationSequenceAxes=FollowerAxes  RotationSequence=XYX  RotationSequenceAngles=[0 0 0]  RotationSequenceAnglesUnits=deg  RotationMatrix=[1 0 0; 0 1 0; 0 0 1]  Quaternion=[1 0 0 0]
  Transform1 : sm_lib/Frames and Transforms/Rigid Transform  TranslationMethod=Cartesian  TranslationStandardOffset=0  TranslationStandardOffsetUnits=mm  TranslationStandardAxis=+Z  TranslationCartesianOffset=[-177.62772197331262 126.39913469758682 -143.11837070913361]  TranslationCartesianOffsetUnits=mm  TranslationROffset=0  TranslationROffsetUnits=m  TranslationZOffset=0  TranslationZOffsetUnits=m  TranslationThetaOffset=0  TranslationThetaOffsetUnits=deg  RotationMethod=ArbitraryAxis  RotationAngleUnits=rad  RotationStandardAxis=+Z  RotationAngle=2.0943951023931953  RotationArbitraryAxis=[0.57735026918962595 0.57735026918962584 0.57735026918962562]  FollAlignAxisA=+X  BaseAlignAxisA=+Y  FollAlignAxisB=+Y  BaseAlignAxisB=+Z  RotationSequenceAxes=FollowerAxes  RotationSequence=XYX  RotationSequenceAngles=[0 0 0]  RotationSequenceAnglesUnits=deg  RotationMatrix=[1 0 0; 0 1 0; 0 0 1]  Quaternion=[1 0 0 0]
  Transform2 : sm_lib/Frames and Transforms/Rigid Transform  TranslationMethod=Cartesian  TranslationStandardOffset=0  TranslationStandardOffsetUnits=mm  TranslationStandardAxis=+Z  TranslationCartesianOffset=[-153.62772197331537 131.82453775326132 -130.4247698928408]  TranslationCartesianOffsetUnits=mm  TranslationROffset=0  TranslationROffsetUnits=m  TranslationZOffset=0  TranslationZOffsetUnits=m  TranslationThetaOffset=0  TranslationThetaOffsetUnits=deg  RotationMethod=ArbitraryAxis  RotationAngleUnits=rad  RotationStandardAxis=+Z  RotationAngle=2.2221940470110662  RotationArbitraryAxis=[0.61437017396793026 -0.61437017396793059 0.49507431631748977]  FollAlignAxisA=+X  BaseAlignAxisA=+Y  FollAlignAxisB=+Y  BaseAlignAxisB=+Z  RotationSequenceAxes=FollowerAxes  RotationSequence=XYX  RotationSequenceAngles=[0 0 0]  RotationSequenceAnglesUnits=deg  RotationMatrix=[1 0 0; 0 1 0; 0 0 1]  Quaternion=[1 0 0 0]
  Transform3 : sm_lib/Frames and Transforms/Rigid Transform  TranslationMethod=Cartesian  TranslationStandardOffset=0  TranslationStandardOffsetUnits=mm  TranslationStandardAxis=+Z  TranslationCartesianOffset=[-167.62772197331242 128.0999109638598 -150.93549038919824]  TranslationCartesianOffsetUnits=mm  TranslationROffset=0  TranslationROffsetUnits=m  TranslationZOffset=0  TranslationZOffsetUnits=m  TranslationThetaOffset=0  TranslationThetaOffsetUnits=deg  RotationMethod=ArbitraryAxis  RotationAngleUnits=rad  RotationStandardAxis=+Z  RotationAngle=1.7850283121554718  RotationArbitraryAxis=[1 8.3181277610745589e-16 -6.6018680201685363e-16]  FollAlignAxisA=+X  BaseAlignAxisA=+Y  FollAlignAxisB=+Y  BaseAlignAxisB=+Z  RotationSequenceAxes=FollowerAxes  RotationSequence=XYX  RotationSequenceAngles=[0 0 0]  RotationSequenceAnglesUnits=deg  RotationMatrix=[1 0 0; 0 1 0; 0 0 1]  Quaternion=[1 0 0 0]
  Transform4 : sm_lib/Frames and Transforms/Rigid Transform  TranslationMethod=Cartesian  TranslationStandardOffset=0  TranslationStandardOffsetUnits=mm  TranslationStandardAxis=+Z  TranslationCartesianOffset=[-167.62772197331242 126.39913469761733 -143.11837070915067]  TranslationCartesianOffsetUnits=mm  TranslationROffset=0  TranslationROffsetUnits=m  TranslationZOffset=0  TranslationZOffsetUnits=m  TranslationThetaOffset=0  TranslationThetaOffsetUnits=deg  RotationMethod=ArbitraryAxis  RotationAngleUnits=rad  RotationStandardAxis=+Z  RotationAngle=1.5707963267948968  RotationArbitraryAxis=[5.5511151231257809e-17 -1 -5.5511151231257809e-17]  FollAlignAxisA=+X  BaseAlignAxisA=+Y  FollAlignAxisB=+Y  BaseAlignAxisB=+Z  RotationSequenceAxes=FollowerAxes  RotationSequence=XYX  RotationSequenceAngles=[0 0 0]  RotationSequenceAnglesUnits=deg  RotationMatrix=[1 0 0; 0 1 0; 0 0 1]  Quaternion=[1 0 0 0]
  joint_1_RIGID : Subsystem
  F2 : PMIOPort  Side=Right
  F1 : PMIOPort  Port=2  Side=Left
  F : PMIOPort  Port=3  Side=Right
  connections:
  Transform/LConn1 -- ReferenceFrame/RConn1 -- Transform3/LConn1 -- Transform4/LConn1 -- Transform2/LConn1 -- Transform1/LConn1
  Transform/RConn1 -- F/RConn1
  Transform1/RConn1 -- F1/RConn1
  Transform2/RConn1 -- F2/RConn1
  Transform3/RConn1 -- joint_1_RIGID/LConn1
  AXE_BRAS_1_RIGID/LConn1 -- Transform4/RConn1

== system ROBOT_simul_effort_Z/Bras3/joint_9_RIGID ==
  AXE_BRAS_1_RIGID : Subsystem
  ReferenceFrame : sm_lib/Frames and Transforms/Reference Frame
  Transform : sm_lib/Frames and Transforms/Rigid Transform  TranslationMethod=Cartesian  TranslationStandardOffset=0  TranslationStandardOffsetUnits=mm  TranslationStandardAxis=+Z  TranslationCartesianOffset=[-181.62772197330938 116.19029839316687 -133.82632242532907]  TranslationCartesianOffsetUnits=mm  TranslationROffset=0  TranslationROffsetUnits=m  TranslationZOffset=0  TranslationZOffsetUnits=m  TranslationThetaOffset=0  TranslationThetaOffsetUnits=deg  RotationMethod=ArbitraryAxis  RotationAngleUnits=rad  RotationStandardAxis=+Z  RotationAngle=1.9754511492118274  RotationArbitraryAxis=[-0.53149434051907796 -0.53149434051907751 -0.65956616953295999]  FollAlignAxisA=+X  BaseAlignAxisA=+Y  FollAlignAxisB=+Y  BaseAlignAxisB=+Z  RotationSequenceAxes=FollowerAxes  RotationSequence=XYX  RotationSequenceAngles=[0 0 0]  RotationSequenceAnglesUnits=deg  RotationMatrix=[1 0 0; 0 1 0; 0 0 1]  Quaternion=[1 0 0 0]
  Transform1 : sm_lib/Frames and Transforms/Rigid Transform  TranslationMethod=Cartesian  TranslationStandardOffset=0  TranslationStandardOffsetUnits=mm  TranslationStandardAxis=+Z  TranslationCartesianOffset=[-188.74209771778101 126.39913469761137 -143.11837070916158]  TranslationCartesianOffsetUnits=mm  TranslationROffset=0  TranslationROffsetUnits=m  TranslationZOffset=0  TranslationZOffsetUnits=m  TranslationThetaOffset=0  TranslationThetaOffsetUnits=deg  RotationMethod=ArbitraryAxis  RotationAngleUnits=rad  RotationStandardAxis=+Z  RotationAngle=2.0943951023931993  RotationArbitraryAxis=[0.57735026918962373 0.57735026918962706 0.57735026918962651]  FollAlignAxisA=+X  BaseAlignAxisA=+Y  FollAlignAxisB=+Y  BaseAlignAxisB=+Z  RotationSequenceAxes=FollowerAxes  RotationSequence=XYX  RotationSequenceAngles=[0 0 0]  RotationSequenceAnglesUnits=deg  RotationMatrix=[1 0 0; 0 1 0; 0 0 1]  Quaternion=[1 0 0 0]
  Transform2 : sm_lib/Frames and Transforms/Rigid Transform  TranslationMethod=Cartesian  TranslationStandardOffset=0  TranslationStandardOffsetUnits=mm  TranslationStandardAxis=+Z  TranslationCartesianOffset=[-153.62772197330932 116.19029839316653 -133.82632242532716]  TranslationCartesianOffsetUnits=mm  TranslationROffset=0  TranslationROffsetUnits=m  TranslationZOffset=0  TranslationZOffsetUnits=m  TranslationThetaOffset=0  TranslationThetaOffsetUnits=deg  RotationMethod=ArbitraryAxis  RotationAngleUnits=rad  RotationStandardAxis=+Z  RotationAngle=1.9754511492118267  RotationArbitraryAxis=[-0.53149434051907773 -0.53149434051907751 -0.6595661695329601]  FollAlignAxisA=+X  BaseAlignAxisA=+Y  FollAlignAxisB=+Y  BaseAlignAxisB=+Z  RotationSequenceAxes=FollowerAxes  RotationSequence=XYX  RotationSequenceAngles=[0 0 0]  RotationSequenceAnglesUnits=deg  RotationMatrix=[1 0 0; 0 1 0; 0 0 1]  Quaternion=[1 0 0 0]
  Transform3 : sm_lib/Frames and Transforms/Rigid Transform  TranslationMethod=Cartesian  TranslationStandardOffset=0  TranslationStandardOffsetUnits=mm  TranslationStandardAxis=+Z  TranslationCartesianOffset=[-167.62772197331239 128.09991096385986 -150.93549038919818]  TranslationCartesianOffsetUnits=mm  TranslationROffset=0  TranslationROffsetUnits=m  TranslationZOffset=0  TranslationZOffsetUnits=m  TranslationThetaOffset=0  TranslationThetaOffsetUnits=deg  RotationMethod=ArbitraryAxis  RotationAngleUnits=rad  RotationStandardAxis=+Z  RotationAngle=1.785028312155472  RotationArbitraryAxis=[1 8.002259724525313e-16 -6.8382944364994947e-16]  FollAlignAxisA=+X  BaseAlignAxisA=+Y  FollAlignAxisB=+Y  BaseAlignAxisB=+Z  RotationSequenceAxes=FollowerAxes  RotationSequence=XYX  RotationSequenceAngles=[0 0 0]  RotationSequenceAnglesUnits=deg  RotationMatrix=[1 0 0; 0 1 0; 0 0 1]  Quaternion=[1 0 0 0]
  Transform4 : sm_lib/Frames and Transforms/Rigid Transform  TranslationMethod=Cartesian  TranslationStandardOffset=0  TranslationStandardOffsetUnits=mm  TranslationStandardAxis=+Z  TranslationCartesianOffset=[-167.62772197331236 126.39913469761737 -143.11837070915064]  TranslationCartesianOffsetUnits=mm  TranslationROffset=0  TranslationROffsetUnits=m  TranslationZOffset=0  TranslationZOffsetUnits=m  TranslationThetaOffset=0  TranslationThetaOffsetUnits=deg  RotationMethod=ArbitraryAxis  RotationAngleUnits=rad  RotationStandardAxis=+Z  RotationAngle=1.5707963267948968  RotationArbitraryAxis=[-0 -1 -0]  FollAlignAxisA=+X  BaseAlignAxisA=+Y  FollAlignAxisB=+Y  BaseAlignAxisB=+Z  RotationSequenceAxes=FollowerAxes  RotationSequence=XYX  RotationSequenceAngles=[0 0 0]  RotationSequenceAnglesUnits=deg  RotationMatrix=[1 0 0; 0 1 0; 0 0 1]  Quaternion=[1 0 0 0]
  joint_1_RIGID : Subsystem
  F2 : PMIOPort  Side=Left
  F : PMIOPort  Port=2  Side=Left
  F1 : PMIOPort  Port=3  Side=Right
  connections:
  Transform/LConn1 -- ReferenceFrame/RConn1 -- Transform3/LConn1 -- Transform4/LConn1 -- Transform2/LConn1 -- Transform1/LConn1
  Transform/RConn1 -- F/RConn1
  Transform1/RConn1 -- F1/RConn1
  Transform2/RConn1 -- F2/RConn1
  Transform3/RConn1 -- joint_1_RIGID/LConn1
  AXE_BRAS_1_RIGID/LConn1 -- Transform4/RConn1
